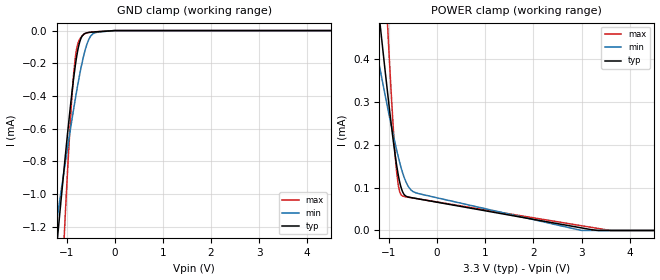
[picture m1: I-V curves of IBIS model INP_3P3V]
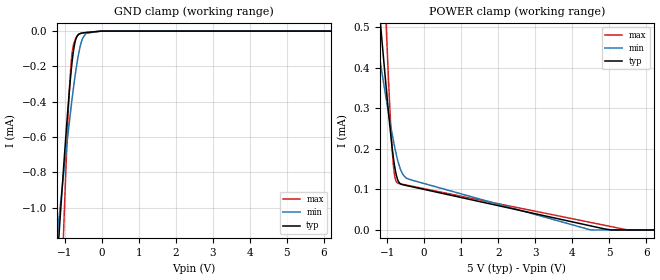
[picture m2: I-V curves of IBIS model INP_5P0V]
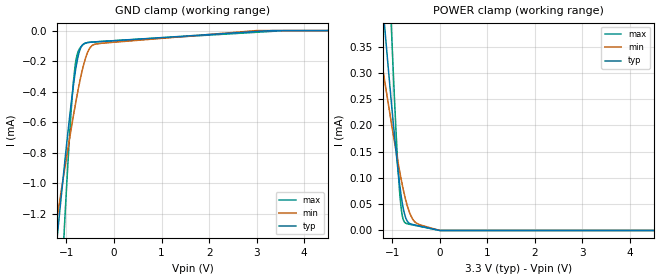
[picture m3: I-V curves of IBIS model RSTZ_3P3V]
| Texas Instruments Incorporated
| 2.5 / 5 A Isolated IGBT Gate Driver with Active Safety Features
| Marketing part#   Voltage Range   Package-type   #pins/pkg drawing
| ISO5852SDW   3.0V - 5.5V   SOIC   16-pin DW
[IBIS Ver]   4.1
[File name]   iso5852s.ibs
[File Rev]   1.0
[Date]   07/31/2015
[Source]   Model built from spectre simulations at:
   Texas Instruments Incorporated.
   Webench Design Center
   12500 TI Blvd
   Dallas, TX -75243
   For Support e-mail: elab_ibis@list.ti.com
[Notes]   Revision History
   Rev 1.0: 07/31/2015
   - Non monotonic behavior result of circuit behavior
   - ccomp values are based on PVT settings:
   MIN: Low Voltage, High Temperature, Weak Process
   TYP: Nominal Voltage, Nominal Temperature, Nominal Process
   MAX: High Voltage, Low Temperature, Fast Process
   - C_comp although listed in numerical order of value are obtained from varying PVT conditions.
   For PVT conditions for each specific value, refer to the buffer description under respective [Model].
   IBIS model user is responsible for using appropriate C_comp to simulate for Signal Integrity.
[Disclaimer]  This model is designed as an aid for customers of Texas Instruments
 TI and its licensors and suppliers make no warranties, either expressed
 or implied, with respect to this  model, including the warranties of
 merchantability or fitness for a particular purpose.
 The model is provided solely on an "as is" basis. The entire risk as to
 its quality and performance is with the customer.
[Copyright] (C)Copyright 2015 Texas Instruments Incorporated.
   All rights reserved.
[Component]   ISO5852SDW
[Manufacturer]  Texas Instruments Incorporated
[Package]   |16-pin SOIC DW package
|   typ   min   max
R_pkg   0.04817   0.03432   0.09530
L_pkg   2.4595nH   1.6904nH   4.7034nH
C_pkg   0.847pF   0.428pF   1.397pF
[Pin]   signal_name   model_name   R_pin   L_pin   C_pin
1   VEE2   GND   0.03455  3.39778n  0.89677p
2   DESAT   NC   0.03432  3.12613n  0.84706p
3   GND2   GND   0.04265  1.85523n  0.57831p
4   NC   NC   0.03948  1.69049n  0.59300p
5   VCC2   POWER   0.03943  1.70546n  0.55709p
6   OUT   NC   0.04257  1.86953n  0.56379p
7   CLAMP   NC   0.04783  1.99000n  0.60148p
8   VEE2   GND   0.03740  4.70338n  1.39696p
9   GND1   GND   0.03763  4.61305n  1.39587p
10   INP   INP   0.08703  5.01514n  1.58483p
11   INN   RSTZ   0.07132  2.45946n  0.43321p
12   RDY   FAULT   0.06147  2.13194n  0.42769p
13   FAULTZ   FAULT   0.07288  2.39260n  0.48001p
14   RSTZ   RSTZ   0.09530  3.03704n  0.47622p
15   VCC1   POWER   0.04817  4.23145n  0.93567p
16   GND1   GND   0.04790  4.51154n  0.99405p
[Model Selector] INP
INP_3P3V   3.3V INPUT
INP_5P0V   5.0V INPUT
[Model Selector] RSTZ
RSTZ_3P3V   3.3V INPUT
RSTZ_5P0V   5.0V INPUT
[Model Selector] FAULT
FAULT_3P3V   3.3V OPEN DRAIN OUTPUT
FAULT_5P0V   5.0V OPEN DRAIN OUTPUT
| Models and submodels in the file (6): INP_3P3V (Input), INP_5P0V (Input), RSTZ_3P3V (Input), RSTZ_5P0V (Input), FAULT_3P3V (Open_drain), FAULT_5P0V (Open_drain)
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|   Model INP_3P3V
[Model]   INP_3P3V
Model_type   Input
Vinl = .99
Vinh = 2.31
|   typ   min   max
|   (nom PVT)   (slow PVT)   (fast PVT)
C_comp   0.02p   0.01p   0.03p
| Where   nom PVT is  Nominal Process, 3.3V, 27C
|   Fast PVT is Strong Process, 3.6V, -40C
|   Slow PVT is Weak Process, 3.0V, 150C
[Model spec]
|subparameter
Vinl   0.99   0.90   1.08
Vinh   2.31   2.10   2.52
[Voltage Range]   3.3   3.0   3.6
[Temperature Range]   27   150   -40
[Power Clamp Reference]   3.3   3.0   3.6
[GND Clamp Reference]   0   0   0
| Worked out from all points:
|   GND clamp passes 1 mA (typ) near -1.10 V on its own axis
[GND Clamp]
|   Voltage   I(typ)   I(min)   I(max)
-3.3V     -8.303mA   -5.636mA   -16.62mA
-1.32V    -1.689mA   -1.404mA   -2.987mA
-1.211V   -1.342mA   -1.18mA    -2.275mA
-1.112V   -1.032mA   -980.4uA   -1.647mA
-1.033V   -790.3uA   -823.2uA   -1.168mA
-904.2mV  -422.8uA   -575.7uA   -477.2uA
-815.1mV  -208.5uA   -414.1uA   -159.4uA
-726mV    -69.53uA   -267.5uA   -53.34uA
-617.1mV  -17.9uA    -123.7uA   -18.77uA
-458.7mV  -9.288uA   -21.06uA   -8.612uA
-3.3mV    -57.95nA   -73.77nA   -54.6nA
6.6V      0A         0A         0A
[POWER Clamp]
|   Voltage   I(typ)   I(min)   I(max)
-3.3V     2.823mA    1.675mA    5.982mA
-1.399V   709.9uA    503uA      1.334mA
-1.31V    614uA      450uA      1.122mA
-1.181V   477.4uA    374.4uA    821uA
-1.082V   374.8uA    317.5uA    595.1uA
-1.013V   305.2uA    278.5uA    442.8uA
-924mV    220.4uA    230.1uA    262.4uA
-844.8mV  154.5uA    189.6uA    140.2uA
-716.1mV  90.08uA    134.3uA    80.57uA
-438.9mV  74.82uA    87.91uA    74.76uA
2.996V    6.068uA    81.43nA    11.17uA
6.6V      0A         0A         0A
|   Model INP_5P0V
[Model]   INP_5P0V
Model_type   Input
Vinl = 1.5
Vinh = 3.5
|   typ   min   max
|   (nom PVT)   (slow PVT)   (fast PVT)
C_comp   0.02p   0.01p   0.03p
| Where   nom PVT is  Nominal Process, 5.0V, 27C
|   Fast PVT is Strong Process, 5.5V, -40C
|   Slow PVT is Weak Process, 4.5V, 150C
[Model spec]
|subparameter
Vinl   1.50   1.35   1.65
Vinh   3.50   3.15   3.85
[Voltage Range]   5.0   4.5   5.5
[Temperature Range]   27   150   -40
[Power Clamp Reference]   5.0   4.5   5.5
[GND Clamp Reference]   0   0   0
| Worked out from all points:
|   GND clamp passes 1 mA (typ) near -1.10 V on its own axis
[GND Clamp]
|   Voltage   I(typ)   I(min)   I(max)
-5V       -14.08mA   -9.34mA    -28.51mA
-1.25V    -1.465mA   -1.26mA    -2.527mA
-1.13V    -1.087mA   -1.016mA   -1.758mA
-1.04V    -811.6uA   -837.1uA   -1.21mA
-1.025V   -766.7uA   -807.6uA   -1.122mA
-890mV    -385.4uA   -549.2uA   -413.2uA
-815mV    -208.3uA   -414uA     -159.1uA
-710mV    -55.07uA   -243.5uA   -45.59uA
-560mV    -12.68uA   -70.43uA   -12.44uA
-425mV    -8.538uA   -15.12uA   -7.899uA
-5mV      -88.08nA   -112.2nA   -82.94nA
10V       0A         0A         0A
[POWER Clamp]
|   Voltage   I(typ)   I(min)   I(max)
-5V       185.7mA    67.09mA    302.4mA
-3.35V    2.914mA    1.745mA    6.164mA
-1.25V    583.9uA    452.7uA    1.016mA
-1.13V    457.8uA    382.9uA    738uA
-1.025V   351uA      323.3uA    503.6uA
-905mV    237.5uA    258.3uA    263.4uA
-830mV    177.9uA    220.7uA    159.8uA
-770mV    143.2uA    193.5uA    123.2uA
-695mV    119.6uA    165.4uA    114.9uA
-410mV    108.3uA    125.1uA    109.4uA
4.495V    10.1uA     112.2nA    18.59uA
10V       0A         0A         0A
|   Model RSTZ_3P3V
[Model]   RSTZ_3P3V
Model_type   Input
Vinl = .99
Vinh = 2.31
|   typ   min   max
|   (nom PVT)   (slow PVT)   (fast PVT)
C_comp   0.02p   0.01p   0.03p
| Where   nom PVT is  Nominal Process, 3.3V, 27C
|   Fast PVT is Strong Process, 3.6V, -40C
|   Slow PVT is Weak Process, 3.0V, 150C
[Model spec]
|subparameter
Vinl   0.99   0.90   1.08
Vinh   2.31   2.10   2.52
[Voltage Range]   3.3   3.0   3.6
[Temperature Range]   27   150   -40
[Power Clamp Reference]   3.3   3.0   3.6
[GND Clamp Reference]   0   0   0
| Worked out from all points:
|   GND clamp passes 1 mA (typ) near -1.08 V on its own axis
[GND Clamp]
|   Voltage   I(typ)   I(min)   I(max)
-3.3V     -8.369mA   -5.712mA   -16.69mA
-1.32V    -1.755mA   -1.48mA    -3.053mA
-1.211V   -1.408mA   -1.257mA   -2.341mA
-1.112V   -1.098mA   -1.057mA   -1.713mA
-1.033V   -856.4uA   -899.5uA   -1.235mA
-904.2mV  -488.8uA   -652uA     -543.8uA
-815.1mV  -274.5uA   -490.5uA   -226uA
-716.1mV  -126.3uA   -328.9uA   -115uA
-597.3mV  -81.53uA   -179.6uA   -82.57uA
-399.3mV  -74.05uA   -88.82uA   -74.04uA
2.996V    -6.069uA   -82.91nA   -11.17uA
6.6V      0A         0A         0A
[POWER Clamp]
|   Voltage   I(typ)   I(min)   I(max)
-3.3V     2.757mA    1.599mA    5.915mA
-1.399V   643.8uA    426.6uA    1.267mA
-1.31V    547.9uA    373.6uA    1.056mA
-1.181V   411.3uA    298.1uA    754.4uA
-1.013V   239.1uA    202.1uA    376.2uA
-924mV    154.4uA    153.7uA    195.7uA
-844.8mV  88.43uA    113.3uA    73.52uA
-785.4mV  50.69uA    85.59uA    27.03uA
-706.2mV  21.73uA    54.52uA    13.5uA
-528mV    10.57uA    16.68uA    9.767uA
-3.3mV    59.22nA    75.71nA    55.66nA
6.6V      0A         0A         0A
